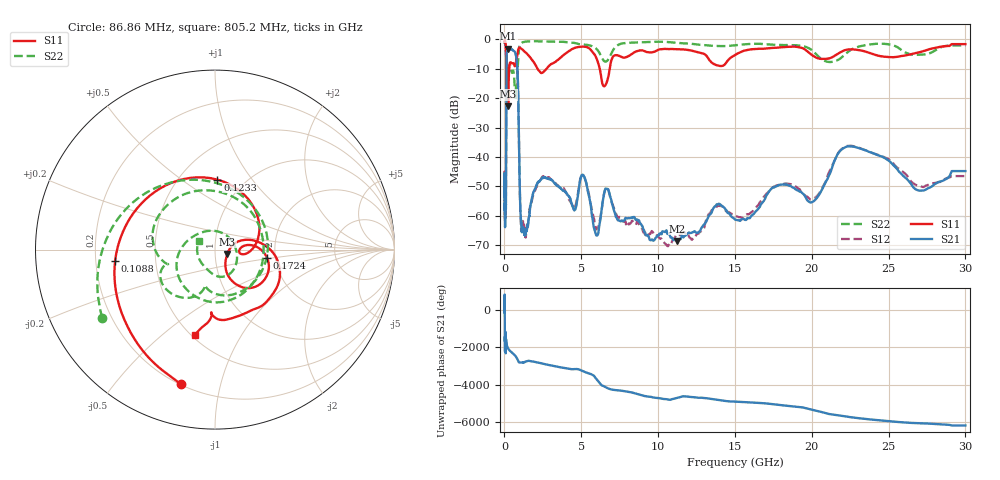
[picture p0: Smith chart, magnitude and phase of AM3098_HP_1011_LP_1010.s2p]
! Date/Time: Thu, Feb 28, 2019 8:43 AM
! Network Analyzer: Agilent Technologies E8364B Rev: A.07.50.67
! Sweep from 0.010 to 30.000 GHz, 1601 Points, Sweep Type: LOG
! Power Supply: 5.023 V, 0.002 A
# Hz S DB R 50
!freq MagS11 AngS11 MagS21 AngS21 MagS12 AngS12 MagS22 AngS22
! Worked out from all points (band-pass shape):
!   1601 points, 10 MHz to 30 GHz, reference 50 ohm
!   highest |S21| = -3.11 dB at 259.9 MHz (marker M1); lowest = -68.7 dB at 11.25 GHz (marker M2)
!   |S21| within 3 dB of the highest: 137.5 MHz to 772.1 MHz (634.6 MHz wide, 140 % of centre)
!   lowest |S11| = -22.7 dB at 242.3 MHz (marker M3), VSWR 1.16, Z = 57.3 - j2.78 ohm
!   |S11| at or under -10 dB: 191.4 MHz to 305.9 MHz (114.5 MHz wide, 46.1 % of centre); 2.156 GHz to 2.738 GHz (582 MHz wide, 23.8 % of centre); 6.204 GHz to 6.849 GHz (645.5 MHz wide, 9.89 % of centre)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
!   |S22| runs from -20.0 to -0.6 dB; largest |S21 - S12| = 0.011
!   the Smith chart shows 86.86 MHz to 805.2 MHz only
!   S11 on the Smith chart (normalised r, x): 86.86 MHz: 0.20, -0.76; 108.8 MHz: 0.28, -0.05; 123.3 MHz: 0.75, +0.69; 172.4 MHz: 1.81, -0.18; 805.2 MHz: 0.52, -0.65
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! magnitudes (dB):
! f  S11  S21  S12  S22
! 10 MHz  -0.3  -46.8  -45.8  -0.6
! 38.04 MHz  -0.4  -60.7  -59.6  -0.9
! 86.86 MHz  -2.2  -55.5  -54.7  -2.7
! 108.8 MHz  -5.0  -35.0  -34.7  -6.3
! 123.3 MHz  -8.2  -14.1  -14.1  -10.6
! 144.7 MHz  -17.2  -5.1  -5.0  -13.7
! 172.4 MHz  -10.6  -4.0  -3.9  -9.7
! 242.3 MHz  -22.7  -3.1  -3.1  -11.2
! 259.9 MHz  -17.8  -3.1  -3.1  -10.9
! 550.5 MHz  -8.1  -3.7  -3.7  -10.6
! 805.2 MHz  -6.2  -7.5  -7.5  -19.8
! 1.098 GHz  -3.1  -63.4  -65.0  -1.2
! 2.084 GHz  -9.3  -49.6  -50.1  -0.6
! 4.525 GHz  -3.0  -58.0  -57.6  -1.1
! 5.103 GHz  -2.4  -46.1  -46.2  -1.7
! 5.929 GHz  -5.7  -66.0  -64.1  -2.9
! 6.653 GHz  -14.6  -50.9  -50.3  -7.4
! 7.926 GHz  -6.0  -60.9  -63.5  -1.2
! 11.25 GHz  -3.3  -68.7  -66.7  -1.2
! 20.1 GHz  -5.6  -55.2  -54.3  -4.1
! 22.56 GHz  -3.4  -36.4  -36.2  -3.5
! 30 GHz  -1.6  -44.8  -46.5  -2.1
